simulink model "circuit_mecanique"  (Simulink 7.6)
settings: Solver=ode15s  StartTime=0.0  StopTime=1.5  RelTol=1e-3
InitFcn:
  |  clc
  | k2=2000;
  | f2=500;
  | m2=10;
  | 
  | m1=5;
  | k1=5000;
  | f1=1000;
StopFcn:
  | close all
  | load pos_vit.mat
  | plotyy(pv(1,:),pv(2,:),pv(1,:),pv(3,:))
  | title('Vitesse et position de la masse 2')
  | xlabel('temps')
  | grid
  | 
  | figure(2)
  | load pos_vit1.mat
  | plotyy(pv1(1,:),pv1(2,:),pv1(1,:),pv1(3,:))
  | title('Vitesse et position de la masse 1')
  | xlabel('temps')
  | grid
libraries: fl_lib x11, nesl_utility x5

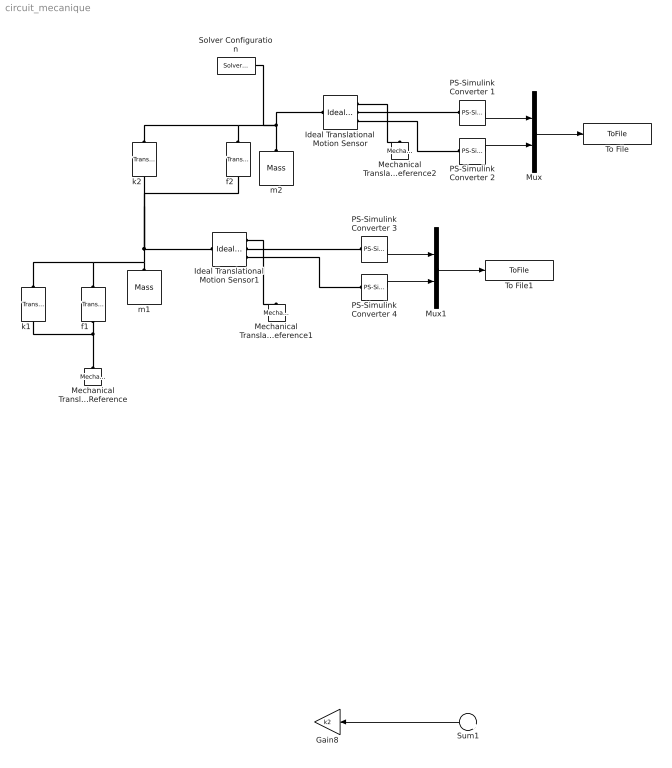
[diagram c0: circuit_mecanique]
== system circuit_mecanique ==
  Gain8 : Gain  Gain=k2
  Ideal Translational Motion Sensor : fl_lib/Mechanical/Mechanical Sensors/Ideal Translational Motion Sensor  DialogController=NetworkEngine.DynNeDlgSource  SystemSampleTime=-1  offset=0 m  v_Log=off  f_Log=off  x_Log=off  LocalVarNames=|v|f|x  LocalVarDescs=|v|f|x  LocalVarLogging=[0 0 0]
  Ideal Translational Motion Sensor1 : fl_lib/Mechanical/Mechanical Sensors/Ideal Translational Motion Sensor  DialogController=NetworkEngine.DynNeDlgSource  SystemSampleTime=-1  offset=0 m  v_Log=off  f_Log=off  x_Log=off  LocalVarNames=|v|f|x  LocalVarDescs=|v|f|x  LocalVarLogging=[0 0 0]
  Mechanical Translational Reference : fl_lib/Mechanical/Translational Elements/Mechanical Translational Reference  DialogController=NetworkEngine.DynNeDlgSource  SystemSampleTime=-1  f_Log=off  LocalVarNames=|f  LocalVarDescs=|f  LocalVarLogging=0
  Mechanical Translational Reference1 : fl_lib/Mechanical/Translational Elements/Mechanical Translational Reference  DialogController=NetworkEngine.DynNeDlgSource  SystemSampleTime=-1  f_Log=off  LocalVarNames=|f  LocalVarDescs=|f  LocalVarLogging=0
  Mechanical Translational Reference2 : fl_lib/Mechanical/Translational Elements/Mechanical Translational Reference  DialogController=NetworkEngine.DynNeDlgSource  SystemSampleTime=-1  f_Log=off  LocalVarNames=|f  LocalVarDescs=|f  LocalVarLogging=0
  Mux : Mux  Inputs=2
  Mux1 : Mux  Inputs=2
  PS-Simulink Converter 1 : nesl_utility/PS-Simulink Converter  DialogController=NetworkEngine.DynNeUtilDlgSource  SystemSampleTime=-1  PhysicalDomain=network_engine_domain  LeftPortType=input  RightPortType=output  SubClassName=ps_output  Unit=m/s  AffineConversion=off
  PS-Simulink Converter 2 : nesl_utility/PS-Simulink Converter  DialogController=NetworkEngine.DynNeUtilDlgSource  SystemSampleTime=-1  PhysicalDomain=network_engine_domain  LeftPortType=input  RightPortType=output  SubClassName=ps_output  Unit=m  AffineConversion=off
  PS-Simulink Converter 3 : nesl_utility/PS-Simulink Converter  DialogController=NetworkEngine.DynNeUtilDlgSource  SystemSampleTime=-1  PhysicalDomain=network_engine_domain  LeftPortType=input  RightPortType=output  SubClassName=ps_output  Unit=m/s  AffineConversion=off
  PS-Simulink Converter 4 : nesl_utility/PS-Simulink Converter  DialogController=NetworkEngine.DynNeUtilDlgSource  SystemSampleTime=-1  PhysicalDomain=network_engine_domain  LeftPortType=input  RightPortType=output  SubClassName=ps_output  Unit=m  AffineConversion=off
  Solver Configuration : nesl_utility/Solver Configuration  DialogController=NetworkEngine.DynNeUtilDlgSource  SystemSampleTime=-1  PhysicalDomain=network_engine_domain  LeftPortType=input  RightPortType=generic  SubClassName=solver  Accelerate=off  Profile=off  ResidualTolerance=1e-9  MaxNonlinIter=12  MaxModeIter=2  DoFixedCost=off  UseLocalSampling=off  DoDC=off  LinearAlgebra=Sparse  LocalSolverSampleTime=.001  LocalSolverChoice=NE_BACKWARD_EULER_ADVANCER  UseLocalSolver=off
  Sum1 : Sum  Inputs=|+-
  To File : ToFile  Filename=pos_vit.mat  MatrixName=pv
  To File1 : ToFile  Filename=pos_vit1.mat  MatrixName=pv1
  f1 : fl_lib/Mechanical/Translational Elements/Translational Damper  DialogController=NetworkEngine.DynNeDlgSource  SystemSampleTime=-1  D=f2 N/(m/s)  f_Log=off  v_Log=off  LocalVarNames=|f|v  LocalVarDescs=|f|v  LocalVarLogging=[0 0]
  f2 : fl_lib/Mechanical/Translational Elements/Translational Damper  DialogController=NetworkEngine.DynNeDlgSource  SystemSampleTime=-1  D=f2 N/(m/s)  f_Log=off  v_Log=off  LocalVarNames=|f|v  LocalVarDescs=|f|v  LocalVarLogging=[0 0]
  k1 : fl_lib/Mechanical/Translational Elements/Translational Spring  DialogController=NetworkEngine.DynNeDlgSource  SystemSampleTime=-1  spr_rate=k1 N/m  init_def=0 m  f_Log=off  v_Log=off  x_Log=off  LocalVarNames=|f|v|x  LocalVarDescs=|f|v|x  LocalVarLogging=[0 0 0]
  k2 : fl_lib/Mechanical/Translational Elements/Translational Spring  DialogController=NetworkEngine.DynNeDlgSource  SystemSampleTime=-1  spr_rate=k2 N/m  init_def=0 m  f_Log=off  v_Log=off  x_Log=off  LocalVarNames=|f|v|x  LocalVarDescs=|f|v|x  LocalVarLogging=[0 0 0]
  m1 : fl_lib/Mechanical/Translational Elements/Mass  DialogController=NetworkEngine.DynNeDlgSource  SystemSampleTime=-1  mass=m1 kg  initial_velocity=1 m/s  f_Log=off  LocalVarNames=|f  LocalVarDescs=|f  LocalVarLogging=0
  m2 : fl_lib/Mechanical/Translational Elements/Mass  DialogController=NetworkEngine.DynNeDlgSource  SystemSampleTime=-1  mass=m2 kg  initial_velocity=10 m/s  f_Log=off  LocalVarNames=|f  LocalVarDescs=|f  LocalVarLogging=0
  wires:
  PS-Simulink Converter 1/1 -> Mux/1
  PS-Simulink Converter 2/1 -> Mux/2
  Mux/1 -> To File/1
  PS-Simulink Converter 3/1 -> Mux1/1
  PS-Simulink Converter 4/1 -> Mux1/2
  Mux1/1 -> To File1/1
  ? -> ?
  ? -> ?
  ? -> ?
  Sum1/1 -> Gain8/1
  Gain8/1 -> ?
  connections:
  f2/LConn1 -- Ideal Translational Motion Sensor/LConn1 -- m2/LConn1 -- Solver Configuration/RConn1 -- k2/LConn1
  Ideal Translational Motion Sensor/RConn3 -- PS-Simulink Converter 2/LConn1
  Ideal Translational Motion Sensor/RConn2 -- PS-Simulink Converter 1/LConn1
  Ideal Translational Motion Sensor/RConn1 -- Mechanical Translational Reference2/LConn1
  f1/LConn1 -- k2/RConn1 -- f2/RConn1 -- m1/LConn1 -- Ideal Translational Motion Sensor1/LConn1 -- k1/LConn1
  f1/RConn1 -- Mechanical Translational Reference/LConn1 -- k1/RConn1
  Ideal Translational Motion Sensor1/RConn1 -- Mechanical Translational Reference1/LConn1
  Ideal Translational Motion Sensor1/RConn2 -- PS-Simulink Converter 3/LConn1
  Ideal Translational Motion Sensor1/RConn3 -- PS-Simulink Converter 4/LConn1
